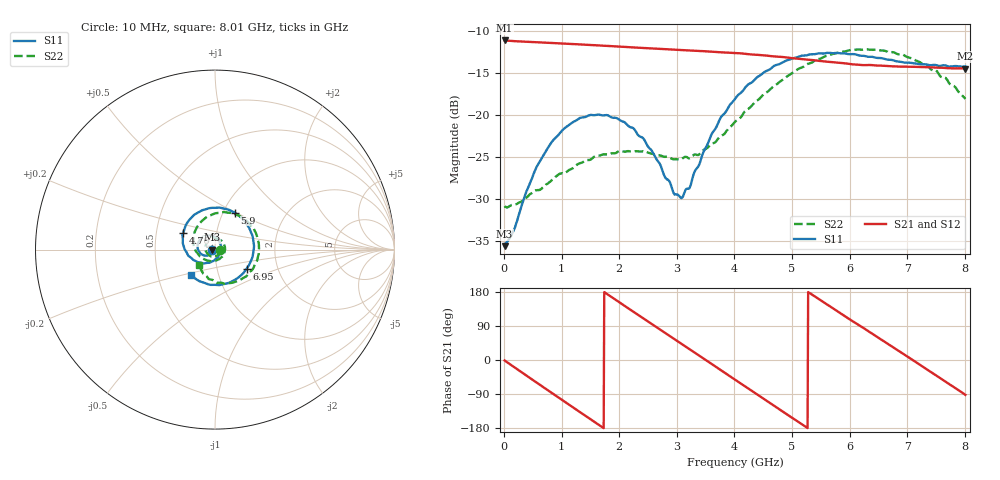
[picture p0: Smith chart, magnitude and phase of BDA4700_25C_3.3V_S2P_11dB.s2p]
!Agilent Technologies,E5071B,MY42404982,A.09.10
!Date: Mon Oct 20 18:07:38 2025
!Data & Calibration Information:
!Freq	S11:SOLT2(ON)	S21:SOLT2(ON)	S12:SOLT2(ON)	S22:SOLT2(ON)
# Hz S RI R 50
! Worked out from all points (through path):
!   801 points, 10 MHz to 8.01 GHz, reference 50 ohm
!   highest |S21| = -11.11 dB at 10 MHz (marker M1); lowest = -14.4 dB at 8.01 GHz (marker M2)
!   group delay of S21, straight-line fit = 281 ps
!   lowest |S11| = -35.6 dB at 10 MHz (marker M3), VSWR 1.03, Z = 48.4 - j0.108 ohm
!   |S11| at or under -10 dB: start of sweep to end of sweep
!   |S22| runs from -31.0 to -12.2 dB; largest |S21 - S12| = 0.0031
!   S11 on the Smith chart (normalised r, x): 10 MHz: 0.97, -0.00; 4.76 GHz: 0.69, +0.13; 5.9 GHz: 1.13, +0.49; 6.95 GHz: 1.39, -0.31; 8.01 GHz: 0.74, -0.22
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1e7  -0.0166 -0.00111  0.2783 -0.00615  0.2781 -0.00628  0.0288 -0.00147
1.6e8  -0.0178 -0.01  0.2635 -0.0814  0.2634 -0.0812  0.0276 -0.00973
3.3e8  -0.0232 -0.0203  0.2245 -0.1571  0.2244 -0.1571  0.0227 -0.0209
7.2e8  -0.0507 -0.0335  0.067 -0.2616  0.0672 -0.2615  -0.00306 -0.0383
1.02e9  -0.0785 -0.0233  -0.0765 -0.2556  -0.0764 -0.2557  -0.0304 -0.0334
1.35e9  -0.0968 0.00741  -0.2039 -0.1668  -0.2038 -0.1668  -0.052 -0.00434
1.93e9  -0.0667 0.0698  -0.2407 0.0893  -0.2407 0.0893  -0.0248 0.054
2.32e9  -0.0174 0.0747  -0.1257 0.2186  -0.1257 0.2187  0.022 0.057
2.68e9  0.0226 0.0478  0.0292 0.2469  0.0287 0.2467  0.053 0.0228
2.95e9  0.0327 0.01  0.1378 0.2034  0.1373 0.2029  0.0534 -0.012
3.09e9  0.0304 -0.011  0.183 0.1619  0.1814 0.1629  0.046 -0.0304
3.54e9  -0.0163 -0.0661  0.239 -0.0164  0.2389 -0.0166  -0.00855 -0.0639
4.01e9  -0.107 -0.0645  0.1451 -0.184  0.1454 -0.1836  -0.0824 -0.0389
4.38e9  -0.1667 -0.00329  0.00252 -0.2287  0.00254 -0.2293  -0.1189 0.0257
4.76e9  -0.1772 0.0936  -0.1377 -0.1752  -0.1368 -0.176  -0.1064 0.1132
5.35e9  -0.0644 0.2213  -0.2107 0.0287  -0.211 0.0275  0.0236 0.2047
5.9e9  0.1107 0.2057  -0.0937 0.1812  -0.0942 0.1803  0.1848 0.1518
6.31e9  0.1981 0.1027  0.0426 0.1943  0.0438 0.1927  0.2445 0.0302
6.68e9  0.2123 -0.0234  0.1482 0.1281  0.1487 0.1278  0.2209 -0.0871
6.95e9  0.1761 -0.1065  0.1884 0.0485  0.1885 0.0472  0.1684 -0.1523
7.47e9  0.029 -0.1971  0.1524 -0.1173  0.1522 -0.1175  0.0137 -0.1854
8.01e9  -0.1343 -0.1417  -0.00639 -0.1895  -0.00584 -0.1896  -0.091 -0.086
